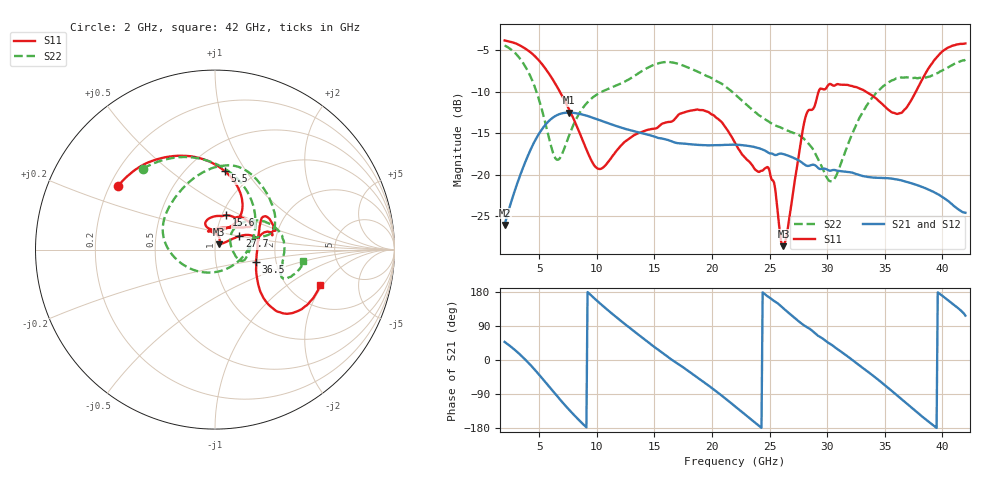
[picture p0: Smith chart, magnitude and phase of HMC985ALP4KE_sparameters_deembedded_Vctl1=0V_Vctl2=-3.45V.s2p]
!s2p File: Measurements: S11, S21, S12, S22
# GHz S dB R 50.0
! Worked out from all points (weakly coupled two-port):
!   401 points, 2 GHz to 42 GHz, reference 50 ohm
!   highest |S21| = -12.49 dB at 7.6 GHz (marker M1); lowest = -26.0 dB at 2 GHz (marker M2)
!   lowest |S11| = -28.6 dB at 26.2 GHz (marker M3), VSWR 1.08, Z = 52.3 + j3.04 ohm
!   |S11| at or under -10 dB: 6.808 GHz to 29.25 GHz (22.44 GHz wide, 124 % of centre); 33.41 GHz to 37.69 GHz (4.28 GHz wide, 12 % of centre)
!   |S22| runs from -20.8 to -4.4 dB; largest |S21 - S12| = 0.00049
!   S11 on the Smith chart (normalised r, x): 2 GHz: 0.23, +0.28; 5.5 GHz: 0.74, +0.80; 15.6 GHz: 1.05, +0.42; 27.7 GHz: 1.30, +0.20; 36.5 GHz: 1.57, -0.23; 42 GHz: 2.94, -1.89
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2  -3.79 146.7  -26.03 47.7  -26.03 47.7  -4.39 131.7
3.6  -4.61 119.6  -19.14 6.9  -19.14 6.9  -6.51 88.1
5.5  -7.11 83.1  -14.03 -57.0  -14.04 -57.0  -13.54 12.0
6.5  -9.24 65.8  -12.83 -93.3  -12.82 -93.3  -18.15 -64.8
7.6  -12.11 53.9  -12.49 -131.4  -12.50 -131.4  -15.23 -142.0
8.7  -15.58 54.4  -12.70 -166.0  -12.70 -166.0  -12.11 -176.0
10.3  -19.29 88.8  -13.44 148.8  -13.42 148.8  -10.08 158.3
12.6  -15.84 109.1  -14.51 91.0  -14.49 91.0  -8.63 124.9
15.4  -14.15 75.4  -15.57 25.6  -15.57 25.6  -6.53 83.7
15.6  -13.90 71.7  -15.60 21.1  -15.61 21.1  -6.47 81.4
19.3  -12.23 33.5  -16.42 -58.3  -16.42 -58.3  -7.88 37.3
22  -16.12 51.6  -16.36 -122.2  -16.38 -122.2  -10.30 15.4
24.9  -19.12 104.4  -17.33 166.4  -17.31 166.4  -13.56 11.3
26.2  -28.60 51.5  -17.50 136.3  -17.52 136.3  -14.45 -4.1
27.7  -16.17 28.8  -18.41 98.0  -18.40 97.9  -15.36 -20.7
28.7  -12.14 12.7  -18.79 77.3  -18.79 77.2  -16.76 -23.1
30.5  -9.22 18.3  -19.42 37.7  -19.43 37.7  -20.69 20.2
33.2  -9.82 34.3  -20.17 -23.3  -20.17 -23.3  -12.17 40.6
35.4  -12.23 11.7  -20.43 -76.3  -20.41 -76.3  -8.80 18.3
36.5  -12.48 -16.6  -20.69 -104.5  -20.70 -104.5  -8.26 6.4
39.5  -5.86 -43.6  -22.25 -179.1  -22.24 -179.2  -7.75 -22.6
42  -4.15 -18.6  -24.57 117.1  -24.56 117.1  -6.12 -7.3
